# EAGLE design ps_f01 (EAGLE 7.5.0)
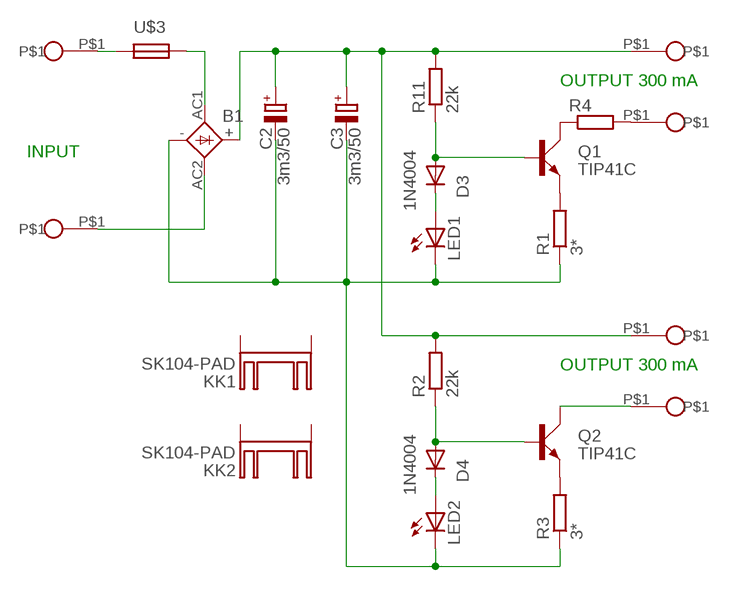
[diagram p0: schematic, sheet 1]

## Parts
B1  SKB  [SKB]
C2  3m3/50  CPOL-EUE7.5-16  [E7,5-16]
C3  3m3/50  CPOL-EUE7.5-16  [E7,5-16]
D3  1N4004  [DO41-10]
D4  1N4004  [DO41-10]
KK1  SK104-PAD  [SK104-PAD]
KK2  SK104-PAD  [SK104-PAD]
LED1  LED5MM  [LED5MM]
LED2  LED5MM  [LED5MM]
Q1  TIP41C  [TO220AV]
Q2  TIP41C  [TO220AV]
R1  3*  R-EU_0207/10  [0207/10]
R2  22k  R-EU_0207/10  [0207/10]
R3  3*  R-EU_0207/10  [0207/10]
R4  R-EU_0414/15  [0414/15]
R11  22k  R-EU_0207/10  [0207/10]
U$1  PIN  [PIN]
U$2  PIN  [PIN]
U$3  FUSEF1  [FUSE]
U$6  PIN  [PIN]
U$7  PIN  [PIN]
U$10  PIN  [PIN]
U$19  PIN  [PIN]

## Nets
GND: B1.- C2.- C3.- LED1.K(C) LED2.K(C) R1.1 R3.1
N$1: R4.2 U$7.P$1
N$2: Q1.E R1.2
N$3: B1.AC2 U$19.P$1
N$4: U$3.P$2 U$10.P$1
N$5: D3.A Q1.B R11.1
N$6: Q1.C R4.1
N$7: D3.C LED1.A
N$8: B1.+ C2.+ C3.+ R2.2 R11.2 U$1.P$1 U$6.P$1
N$13: Q2.E R3.2
N$14: Q2.C U$2.P$1
N$15: D4.A Q2.B R2.1
N$16: D4.C LED2.A
N$19: B1.AC1 U$3.P$4
Unconnected: KK1.K1(K) KK1.K2(K) KK2.K1(K) KK2.K2(K)

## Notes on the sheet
- OUTPUT 300 mA
- INPUT
- OUTPUT 300 mA

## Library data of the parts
B1 = rectifier:SKB: SEMIKRON RECTIFIER
C2 C3 = rcl:CPOL-EU: POLARIZED CAPACITOR, European symbol
D3 D4 = diode:1N4004: DIODE
KK1 KK2 = heatsink:SK104-PAD: HEATSINK
LED1 LED2 = led:LED: LED
Q1 Q2 = transistor-power:TIP41C: NPN TRANSISTOR
R1-R4 R11 = rcl:R-EU_: RESISTOR, European symbol
U$1 U$2 U$6 U$7 U$10 U$19 = LAMPY02:PIN
U$3 = lampy03:FUSE

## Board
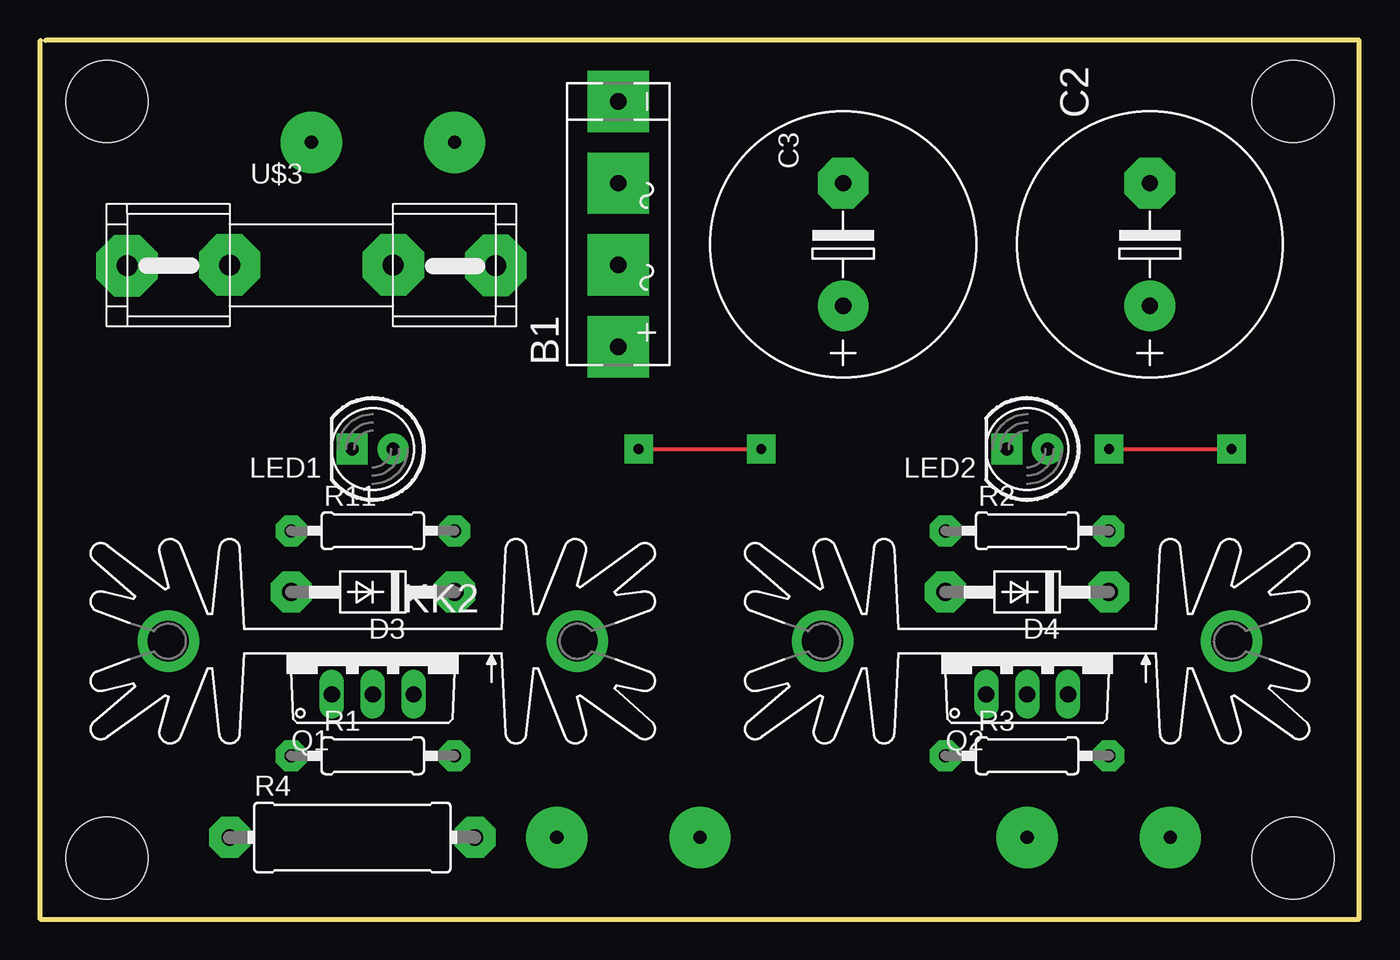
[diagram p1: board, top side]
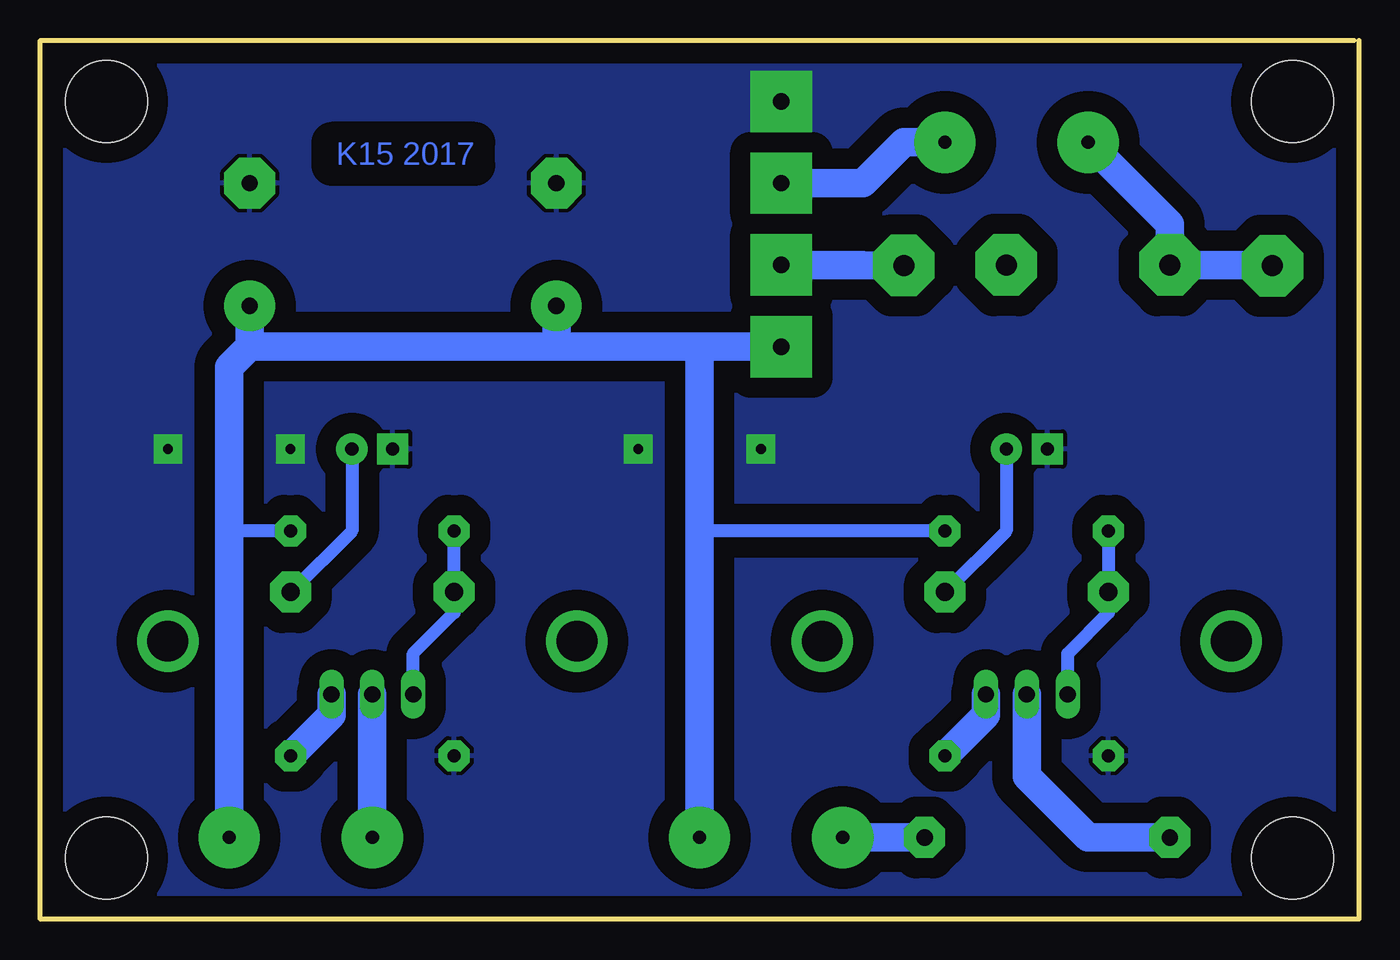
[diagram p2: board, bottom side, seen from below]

Size 81.92 x 54.6 mm. Coordinates in mm from the lower left corner, seen from the top.
Outline: 0.33,54.6 81.92,54.6 81.92,0 0,0 0,54.6
Copper layers (1*16): Top 0.035mm / dielectric 1.5mm / Bottom 0.035mm
Design rules "default": minimum track width 10mil, minimum drill 24mil, track to track 8mil, track to pad 8mil, pad to pad 8mil, via to via 8mil, smd to smd 8mil, copper to edge 40mil, drill to drill 8mil, minimum pad ring 10mil, minimum via ring 8mil, stop-mask expansion 4mil, vias tented up to drill 0mil, thermal gap 10mil
Holes 5.08 mm at 4.14,3.81 77.8,3.81 4.14,50.8 77.8,50.8

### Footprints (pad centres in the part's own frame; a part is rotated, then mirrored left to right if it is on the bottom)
SKB = drill 1.016 long: + -7.62,0; - 7.62,0; AC1 -2.54,0; AC2 2.54,0
E7,5-16 = drill 1.016 pad 3.15: + -3.81,0 | drill 1.016 pad 3.15 octagon: - 3.81,0
DO41-10 = drill 1.118 pad 2.54 octagon: A 5.08,0; C -5.08,0
SK104-PAD = drill 2.54 pad 3.81: K1 -12.7,-0.762; K2 12.7,-0.762
LED5MM = drill 0.813 pad 1.93: A -1.27,0 | drill 0.813 pad 1.93 square: K 1.27,0
TO220AV = drill 1.016 long: B -2.54,-2.54; C 0,-2.54; E 2.54,-2.54
0207/10 = drill 0.813 pad 1.93 octagon: 1 -5.08,0; 2 5.08,0
0414/15 = drill 1.016 pad 2.54 octagon: 1 -7.62,0; 2 7.62,0
PIN = drill 0.813 pad 3.81: P$1 0,0
FUSE = drill 1.3 pad 3.81 octagon: P$1 -5.08,0; P$2 -11.448,-0.051; P$3 5.08,0; P$4 11.448,-0.025

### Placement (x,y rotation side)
B1  35.89,43.18 90 top
C2  68.91,41.91 90 top
C3  49.86,41.91 90 top
D3  20.65,20.32 180 top
D4  61.29,20.32 180 top
KK1  61.29,16.51 180 top
KK2  20.65,16.51 180 top
LED1  20.65,29.21 180 top
LED2  61.29,29.21 180 top
Q1  20.65,16.51 0 top
Q2  61.29,16.51 0 top
R1  20.65,10.16 0 top
R2  61.29,24.13 0 top
R3  61.29,10.16 0 top
R4  19.38,5.08 0 top
R11  20.65,24.13 0 top
U$1  40.97,5.08 0 top
U$2  61.29,5.08 0 top
U$3  16.84,40.64 0 top
U$6  70.18,5.08 0 top
U$7  32.08,5.08 0 top
U$10  16.84,48.26 90 top
U$19  25.73,48.26 90 top

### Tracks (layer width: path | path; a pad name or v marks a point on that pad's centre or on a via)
GND  (via drill 0.6 pad 1.78, 0.6 pad 3.81)
  Top 0.254: v37.16,29.21 v44.78,29.21 | v66.37,29.21 v73.99,29.21
  other vias: 35.89,50.8
  pour Bottom (isolate 1.27): 0.33,54.61 81.61,54.61 81.61,0 0.33,0
N$1
  Bottom 1.778: R4.2 U$7.P$1
N$2
  Bottom 1.778: Q1.E 23.19,12.7 R1.2
N$3
  Bottom 1.778: B1.AC2 30.81,45.72 28.27,48.26 U$19.P$1
N$4
  Bottom 1.778: U$10.P$1 11.76,43.18 11.76,40.64 5.44,40.64 U$3.P$2
N$5
  Bottom 0.813: R11.1 D3.A 15.57,19.05 18.11,16.51 Q1.B
N$6
  Bottom 1.778: R4.1 16.84,5.08 20.65,8.89 Q1.C
N$7
  Bottom 0.813: LED1.A 21.92,24.13 D3.C
N$8  (via drill 0.6 pad 3.81)
  Bottom 0.813: R2.2 70.18,24.13 | R11.2 40.97,24.13
  Bottom 1.778: B1.+ 40.97,35.56 | 40.97,35.56 49.86,35.56 | 49.86,35.56 68.91,35.56 | 68.91,35.56 C2.+ | C3.+ 49.86,35.56 | U$6.P$1 70.18,24.13 70.18,34.29 68.91,35.56 | U$1.P$1 40.97,24.13 40.97,35.56
  other vias: 35.89,35.56
N$9  (via drill 0.6 pad 3.81)
  other vias: 35.89,45.72
N$10  (via drill 0.6 pad 3.81)
  other vias: 35.89,40.64
N$13
  Bottom 1.778: Q2.E 63.83,12.7 R3.2
N$14
  Bottom 1.778: U$2.P$1 Q2.C
N$15
  Bottom 0.813: Q2.B 58.75,16.51 56.21,19.05 D4.A R2.1
N$16
  Bottom 0.813: LED2.A 62.56,24.13 D4.C
N$19
  Bottom 1.778: B1.AC1 30.85,40.64 U$3.P$4

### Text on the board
Bottom: K15 2017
